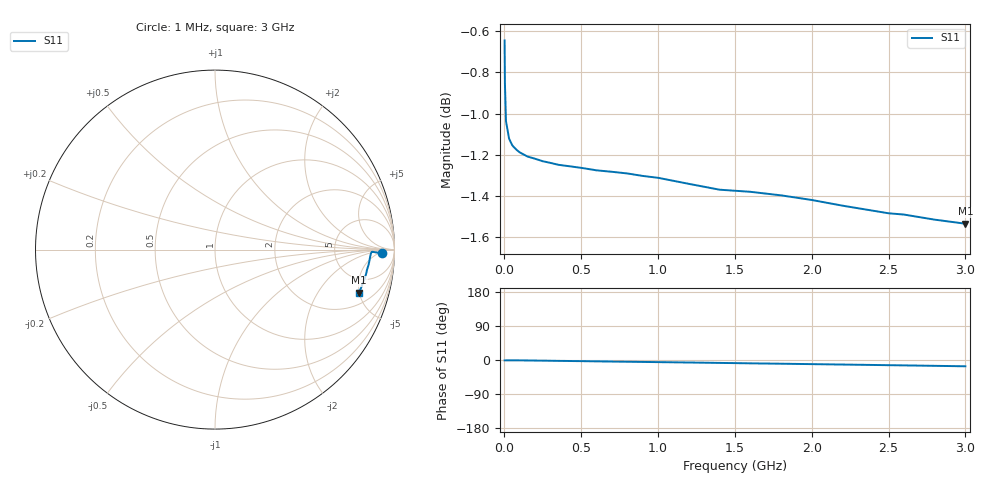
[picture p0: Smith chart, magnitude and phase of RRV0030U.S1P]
! SIEMENS Small Signal Semiconductors
! BA595
! Si PIN Diode in SOD323
! IF = 0.03 mA
! S-Parameters:  July  1992
# GHz  S  MA  R  50
!  f  S11
! GHz  MAG  ANG
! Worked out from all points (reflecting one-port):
!   33 points, 1 MHz to 3 GHz, reference 50 ohm
!   lowest |S11| = -1.5 dB at 3 GHz (marker M1), VSWR 11.35, Z = 155 - j249 ohm
!   phase of S11 starts at -1 deg and turns -16 deg over the sweep
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0.001  0.9285 -1.1
0.003  0.9067 -1.1
0.01  0.8875 -0.9
0.03  0.8789 -0.8
0.05  0.8757 -0.8
0.06  0.8748 -0.9
0.08  0.8733 -0.9
0.15  0.8701 -1.2
0.2  0.869 -1.5
0.25  0.8678 -1.7
0.35  0.8661 -2.3
0.4  0.8656 -2.5
0.45  0.8651 -2.8
0.5  0.8646 -3.0
0.6  0.8634 -3.6
0.8  0.8619 -4.6
1  0.8598 -5.6
1.2  0.8569 -6.6
1.4  0.8541 -7.7
1.5  0.8536 -8.2
1.6  0.8531 -8.8
1.8  0.8514 -9.8
2  0.8492 -10.9
2.4  0.8441 -13.1
2.5  0.8429 -13.7
2.6  0.8423 -14.2
2.8  0.8399 -15.4
3  0.838 -16.6
